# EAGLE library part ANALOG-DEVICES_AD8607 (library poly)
Precision Micropower, Low Noise CMOS, Rail-to-Rail Input/Output Operational Amplifiers Source: http://www.analog.com/static/imported-files/data_sheets/AD8603_8607_8609.pdf
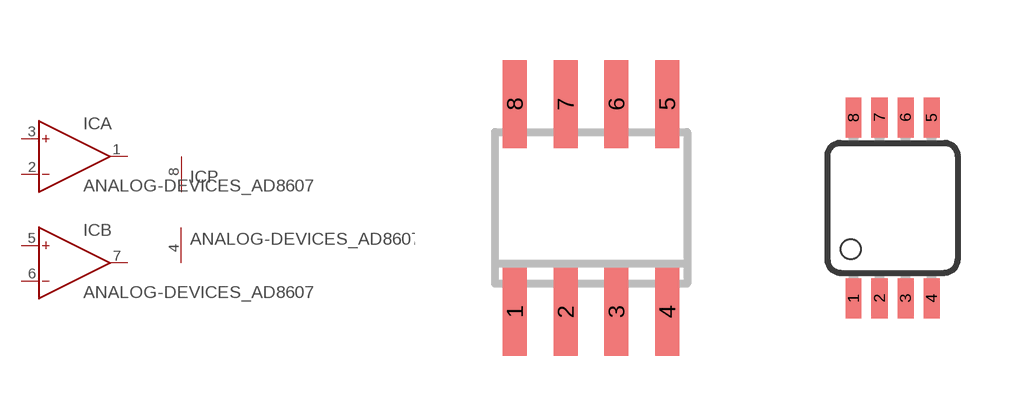
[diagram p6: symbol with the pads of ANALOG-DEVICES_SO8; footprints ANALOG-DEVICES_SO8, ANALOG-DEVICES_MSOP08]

Designator prefix IC; gates A=ANALOG-DEVICES_OP B=ANALOG-DEVICES_OP P=ANALOG-DEVICES_PWR+-

## ANALOG-DEVICES_AD8607R (MPN: AD8607ARMZ-R2; OC_FARNELL: 1651293; OC_NEWARK: 19M8927)  [ANALOG-DEVICES_SO8]
1  A:OUT  out
2  A:IN-  in
3  A:IN+  in
4  P:V-  pwr
5  B:IN+  in
6  B:IN-  in
7  B:OUT  out
8  P:V+  pwr

## ANALOG-DEVICES_AD8607RM (MF: ALTERA CORPORATION; MPN: AD8607ARMZ-REEL; OC_FARNELL: 1464990; OC_NEWARK: 59K6925)  [ANALOG-DEVICES_MSOP08]
Pads as for ANALOG-DEVICES_SO8

## Footprint ANALOG-DEVICES_SO8 (pad centres in mm)
8-Lead Small Outline IC (SO-8) Source: http://www.analog.com/UploadedFiles/Data_Sheets/703465986AD8611_2_0.pdf
smd 0.6 x 2.2: 1 -1.905,-2.6; 2 -0.635,-2.6; 3 0.635,-2.6; 4 1.905,-2.6; 5 1.905,2.6; 6 0.635,2.6; 7 -0.635,2.6; 8 -1.905,2.6

## Footprint ANALOG-DEVICES_MSOP08 (pad centres in mm)
8-Lead micro SO (RM-8) Source: http://www.analog.com/UploadedFiles/Data_Sheets/703465986AD8611_2_0.pdf
smd 0.4 x 1: 1 -0.976,-2.263; 2 -0.326,-2.263; 3 0.324,-2.263; 4 0.974,-2.263; 5 0.974,2.262; 6 0.324,2.262; 7 -0.326,2.262; 8 -0.976,2.262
